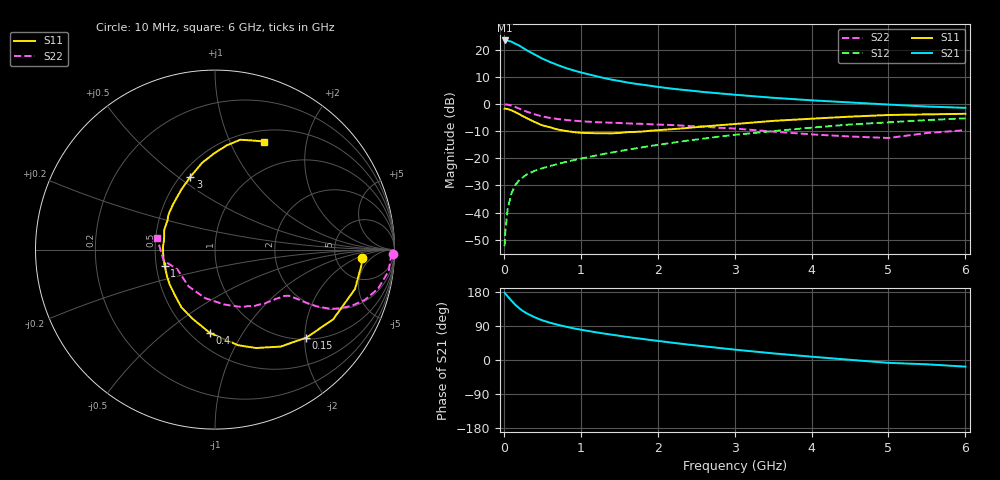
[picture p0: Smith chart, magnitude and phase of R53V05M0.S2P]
! SIEMENS Small Signal Semiconductors
! BFR183
! Si NPN RF Bipolar Junction Transistor in SOT23
! VCE = 3 V  IC = 5 mA
! Common Emitter S-Parameters:  May  1996
# GHz  S  MA  R  50
!  f  S11  S21  S12  S22
! GHz  MAG  ANG  MAG  ANG  MAG  ANG  MAG  ANG
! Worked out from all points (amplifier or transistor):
!   36 points, 10 MHz to 6 GHz, reference 50 ohm
!   highest |S21| = 23.4 dB at 10 MHz (marker M1)
!   |S21| within 3 dB of that: start of sweep to 263.1 MHz
!   unconditionally stable (mu >= 1): 1.027 GHz to 2.639 GHz
!   at 250 MHz: K = 0.42, MSG = 23.8 dB, |S12| = -27.0 dB
!   at 1.4 GHz: K = 1.06, MAG = 11.9 dB, |S12| = -17.9 dB
!   at 6 GHz: K = 0.88, MSG = 1.9 dB, |S12| = -5.3 dB
!   lowest NFmin = 1.15 dB at 450 MHz
!   S11 on the Smith chart (normalised r, x): 10 MHz: 9.42, -2.75; 150 MHz: 1.04, -2.03; 400 MHz: 0.62, -0.73; 1 GHz: 0.55, -0.11; 3 GHz: 0.56, +0.56; 6 GHz: 0.63, +1.35
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0.01  0.8219 -3.3  14.85 177.7  0.0024 93.6  0.9904 -1.4
0.02  0.8205 -6.1  14.65 174.9  0.0046 89.9  0.9797 -2.8
0.05  0.8104 -15.7  14.73 167.8  0.0118 81.4  0.9752 -7.0
0.1  0.7645 -30.5  14.06 156.3  0.0228 74.8  0.9346 -13.4
0.15  0.7068 -44.0  12.93 145.4  0.0322 68.8  0.8815 -18.5
0.2  0.6519 -56.0  11.96 136.6  0.0396 64.7  0.823 -22.4
0.25  0.5939 -67.4  10.79 129.0  0.0449 60.8  0.7664 -25.3
0.3  0.5482 -76.4  9.764 122.8  0.0506 58.6  0.7221 -27.2
0.4  0.4663 -93.3  8.187 112.9  0.0587 56.1  0.6468 -29.2
0.5  0.405 -108.0  6.885 104.6  0.0654 55.6  0.5909 -30.2
0.6  0.3722 -120.1  5.948 98.4  0.0721 55.2  0.5551 -30.7
0.8  0.3197 -141.7  4.642 88.3  0.0853 55.9  0.5107 -31.4
1  0.2947 -161.6  3.828 80.0  0.0983 57.6  0.482 -32.2
1.1  0.2918 -169.4  3.53 76.6  0.1054 58.0  0.4725 -33.1
1.3  0.2901 176.5  3.018 69.9  0.1204 58.8  0.457 -34.6
1.6  0.3031 159.1  2.504 60.9  0.1434 58.6  0.4402 -38.2
2.2  0.3449 132.3  1.909 45.4  0.1942 56.9  0.4097 -47.2
3  0.4279 108.8  1.485 27.4  0.2701 50.8  0.3538 -64.9
3.5  0.4891 98.4  1.303 17.5  0.3168 45.4  0.3101 -80.5
4.5  0.5851 83.5  1.07 0.5  0.4193 33.4  0.2522 -125.8
5.5  0.6444 70.5  0.9 -11.4  0.5065 21.0  0.2925 -168.1
6  0.6612 65.5  0.851 -17.5  0.5458 12.7  0.3292 168.7
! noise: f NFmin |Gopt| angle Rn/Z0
0.45  1.15  0.25  40  0.26
0.9  1.2  0.25  93  0.22
1.8  1.95  0.32  170  0.13
